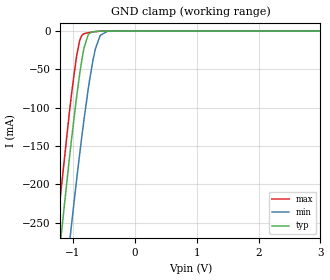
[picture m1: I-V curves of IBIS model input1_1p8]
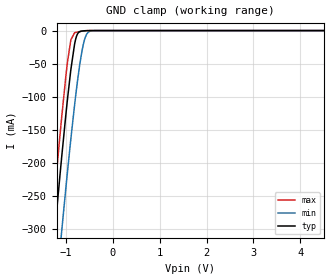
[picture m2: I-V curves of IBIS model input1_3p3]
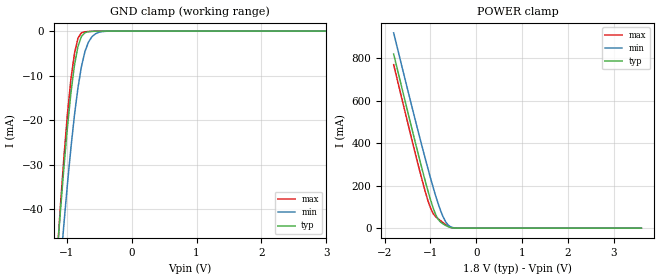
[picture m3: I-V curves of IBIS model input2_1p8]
| Texas Instruments Incorporated
| TLV320ADC5120 2-Channel, 768-kHz, Burr-Brown Audio ADC
[IBIS Ver]   4.1
[File name]   tlv320adc5120.ibs
[Date]   03/03/2021
[File Rev]   1.0
[Source]
| Texas Instruments Incorporated.
| PADC, ASC
| TI India
| Bangalore
[Notes]   Revision History:
| Rev 1.0: 03/03/2021
| - Initial version of the model
| - Model generated from simulations in SPECTRE
| - C_comp although listed in numerical order of value are
|   obtained from varying PVT conditions. For PVT conditions for
|   each specific value refer the buffer description under
|   respective [Model]. IBIS model user is responsible for using
|   appropriate C_comp to simulate for Signal Integrity.
| - Warnings regarding combined Non-monotonicity of various models have been
|   reviewd and considered minor and can be ignored.
| - Model names with a trailing _1p8 contain the model for 1.8V operation.
|   Model names with a trailing _3p3 contain the model for 3.3V operation.
[Disclaimer]
| This model is designed as an aid for customers of Texas Instruments.
| TI and its licensors and suppliers make no warranties, either expressed
| or implied, with respect to this  model, including the warranties of
| merchantability or fitness for a particular purpose. The model is
| provided solely on an "as is" basis. The entire risk as to its quality
| and performance is with the customer.
| This model is subject to change without notice. Texas Instruments
| Incorporated is not responsible for updating this model.
[Copyright]
(C) Copyright 2021 Texas Instruments Incorporated.All rights reserved.
|  Component TLV320ADC5120RTE 20-Pin WQFN - RTE package
|  Part # TLV320ADC5120RTE
[Component]   TLV320ADC5120RTE
[Manufacturer]  TI
[Package]   |20 WQFN - RTE package
|   typ   min   max
R_pkg   0.05   0.04   0.06
L_pkg   1.0nH   0.8nH   1.2nH
C_pkg   0.2pF   0.16pF   0.24pF
[Pin]  signal_name   model_name   R_pin   L_pin   C_pin
1   IN1P   nc   NA   NA   NA
2   IN1M   nc   NA   NA   NA
3   IN2P_GPI1   input1   NA   NA   NA
4   IN2M_GPO1   output   NA   NA   NA
5   VSS   gnd   NA   NA   NA
6   SDOUT   io   NA   NA   NA
7   BCLK   io   NA   NA   NA
8   FSYNC   io   NA   NA   NA
9   IOVDD   power   NA   NA   NA
10   VSS   gnd   NA   NA   NA
11   GPIO1   io   NA   NA   NA
12   SDA   od   NA   NA   NA
13   SCL   od   NA   NA   NA
14   DREG   power   NA   NA   NA
15   VSS   gnd   NA   NA   NA
16   AVDD   power   NA   NA   NA
17   AREG   power   NA   NA   NA
18   VREF   nc   NA   NA   NA
19   MICBIAS_GPI2  input2   NA   NA   NA
20   VSS   gnd   NA   NA   NA
|   Model Selectors
[Model Selector] input1
input1_1p8   1.8V   digital Input
input1_3p3   3.3V   digital Input
[Model Selector] input2
input2_1p8   1.8V   digital Input
input2_3p3   3.3V   digital Input
[Model Selector] output
output_1p8   1.8V   digital Output
output_3p3   3.3V   digital Output
[Model Selector] io
io_1p8   1.8V   digital I/O
io_3p3   3.3V   digital I/O
[Model Selector] od
od_1p8   1.8V   digital I/O Open-drain
od_3p3   3.3V   digital I/O Open-drain
| Models and submodels in the file (10): input1_1p8 (Input), input1_3p3 (Input), input2_1p8 (Input), input2_3p3 (Input), output_1p8 (3-state), output_3p3 (3-state), io_1p8 (I/O), io_3p3 (I/O), od_1p8 (I/O_open_drain), od_3p3 (I/O_open_drain)
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|   input1_1p8 Model
[Model]   input1_1p8
Model_type   Input
Vinl = 0.63
Vinh = 1.17
|   typ   min   max
C_comp   0.9411pF   0.9029pF   0.9992pF
[Model spec]
|subparameter
Vinl   0.63   0.567   0.693
Vinh   1.17   1.053   1.287
| Where Nom  PVT is Nominal Process, 1.8V, 27C
|   Fast PVT is Strong Process,  1.98V, -40C
|   Slow PVT is Weak Process,   1.62V, 150C
[Voltage Range]   1.8   1.62   1.98
|Junction Temperature
[Temperature Range]   27   150   -40
[Power Clamp Reference]   1.8   1.62   1.98
[GND Clamp Reference]   0   0   0
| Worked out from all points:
|   GND clamp passes 1 mA (typ) near -0.68 V on its own axis
[GND Clamp]
|   Voltage   I(typ)   I(min)   I(max)
-1.8V     -769.4mA   -875.1mA   -713.6mA
-1.465V   -489.2mA   -598.8mA   -430.8mA
-1.228V   -297mA     -409mA     -236.8mA
-1.206V   -280mA     -392.1mA   -219.8mA
-1.028V   -146mA     -257.5mA   -86.9mA
-892.8mV  -58.07mA   -162.7mA   -13.59mA
-817.2mV  -21.36mA   -114.1mA   -3.368mA
-747mV    -4.455mA   -73.31mA   -2.124mA
-633.6mV  -487.8uA   -22.64mA   -682.1uA
-558mV    -119.9uA   -5.685mA   -166.1uA
-444.6mV  -3.707uA   -331.7uA   -2.899uA
3.6V      0A         0A         0A
[POWER Clamp]
|   Voltage   I(typ)   I(min)   I(max)
-1.8V     0A         0A         0A
0V        0A         0A         0A
3.6V      0A         0A         0A
|   input1_3p3 Model
[Model]   input1_3p3
Model_type   Input
Vinl = 0.8
Vinh = 2
|   typ   min   max
C_comp   0.8273pF   0.7974pF   0.8702pF
| Where Nom  PVT is Nominal Process, 3.3V, 27C
|   Fast PVT is Strong Process,  3.6V, -40C
|   Slow PVT is Weak Process,   3.0V, 150C
[Voltage Range]   3.3   3   3.6
|Junction Temperature
[Temperature Range]   27   150   -40
[Power Clamp Reference]   3.3   3   3.6
[GND Clamp Reference]   0   0   0
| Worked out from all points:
|   GND clamp passes 1 mA (typ) near -0.68 V on its own axis
[GND Clamp]
|   Voltage   I(typ)   I(min)   I(max)
-3.3V     -2.018A    -2.043A    -2.005A
-1.31V    -362.7mA   -474mA     -303.1mA
-1.261V   -323.1mA   -434.8mA   -263.2mA
-1.201V   -276.3mA   -388.4mA   -216mA
-1.092V   -193mA     -305.2mA   -132.8mA
-963.6mV  -101.9mA   -211.4mA   -46.17mA
-894.3mV  -58.92mA   -163.7mA   -14.05mA
-815.1mV  -20.57mA   -112.8mA   -3.303mA
-745.8mV  -4.323mA   -72.66mA   -2.107mA
-636.9mV  -514.1uA   -23.73mA   -714.4uA
-468.6mV  -8.691uA   -624.3uA   -8.339uA
6.6V      0A         0A         0A
[POWER Clamp]
|   Voltage   I(typ)   I(min)   I(max)
-3.3V     0A         0A         0A
0V        0A         0A         0A
6.6V      0A         0A         0A
|   input2_1p8 Model
[Model]   input2_1p8
Model_type   Input
Vinl = 0.63
Vinh = 1.17
|   typ   min   max
C_comp   5.1126pF   5.054pF   5.172pF
[Model spec]
|subparameter
Vinl   0.63   0.567   0.693
Vinh   1.17   1.053   1.287
| Where Nom  PVT is Nominal Process, 1.8V, 27C
|   Fast PVT is Strong Process,  1.98V, -40C
|   Slow PVT is Weak Process,   1.62V, 150C
[Voltage Range]   1.8   1.62   1.98
|Junction Temperature
[Temperature Range]   27   150   -40
[Power Clamp Reference]   1.8   1.62   1.98
[GND Clamp Reference]   0   0   0
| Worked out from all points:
|   GND clamp passes 1 mA (typ) near -0.76 V on its own axis
|   POWER clamp passes 1 mA (typ) near -0.50 V on its own axis
[GND Clamp]
|   Voltage   I(typ)   I(min)   I(max)
-1.8V     -193.9mA   -198.2mA   -213.1mA
-1.152V   -50.85mA   -62.6mA    -51.1mA
-1.098V   -40.39mA   -52.74mA   -39.26mA
-1.044V   -30.55mA   -43.3mA    -28.29mA
-990mV    -21.58mA   -34.4mA    -18.62mA
-936mV    -13.84mA   -26.19mA   -10.78mA
-882mV    -7.698mA   -18.9mA    -5.071mA
-828mV    -3.464mA   -12.75mA   -1.59mA
-774mV    -1.182mA   -7.957mA   -368.1uA
-666mV    -128.6uA   -2.474mA   -94.52uA
-450mV    -11.5uA    -107.3uA   -13.31uA
3.6V      0A         0A         0A
[POWER Clamp]
|   Voltage   I(typ)   I(min)   I(max)
-1.8V     819.8mA    919.7mA    770mA
-1.314V   391.2mA    496.3mA    339.1mA
-1.152V   254.5mA    360.6mA    203.9mA
-1.044V   168.7mA    273.3mA    123.7mA
-990mV    129mA      230.7mA    91.11mA
-936mV    93mA       189.6mA    67.42mA
-828mV    40.8mA     113.8mA    43.61mA
-720mV    19.7mA     52.22mA    25.12mA
-612mV    7.131mA    14.49mA    8.525mA
-504mV    990.6uA    2.376mA    745.7uA
-342mV    6.316uA    88.51uA    609.3nA
3.6V      0A         0A         0A
